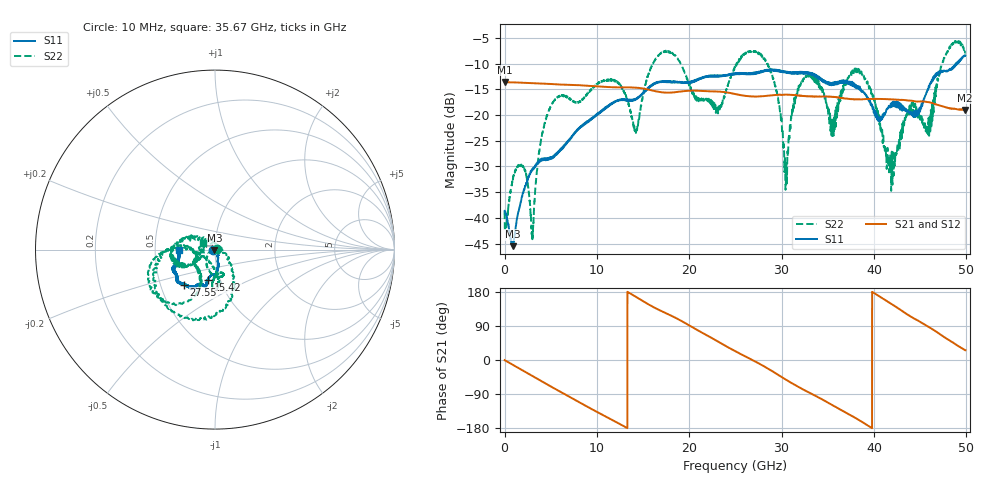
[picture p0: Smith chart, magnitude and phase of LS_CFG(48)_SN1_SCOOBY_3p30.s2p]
!Keysight Technologies,N5245B,MY58422026,A.13.80.08
!Date: Thursday, March 19, 2020 23:41:55
!Correction: S11(Full 2 Port(1,2))
!S21(Full 2 Port(1,2))
!S12(Full 2 Port(1,2))
!S22(Full 2 Port(1,2))
!S2P File: Measurements: S11, S21, S12, S22:
# Hz S DB R 50.0
!freq dBS11 angS11 dBS21 angS21 dBS12 angS12 dBS22 angS22
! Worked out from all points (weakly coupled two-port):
!   4991 points, 10 MHz to 49.91 GHz, reference 50 ohm
!   highest |S21| = -13.58 dB at 10 MHz (marker M1); lowest = -19.0 dB at 49.82 GHz (marker M2)
!   lowest |S11| = -45.5 dB at 870 MHz (marker M3), VSWR 1.01, Z = 49.7 - j0.416 ohm
!   |S11| at or under -10 dB: start of sweep to 48.89 GHz; 48.93533 GHz to 48.99183 GHz (56.5 MHz wide, 0.115 % of centre)
!   |S22| runs from -44.2 to -5.5 dB; largest |S21 - S12| = 0.002
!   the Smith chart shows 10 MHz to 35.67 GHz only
!   S11 on the Smith chart (normalised r, x): 10 MHz: 0.98, -0.01; 15.42 GHz: 0.87, -0.31; 27.55 GHz: 0.66, -0.28; 35.67 GHz: 0.67, -0.00
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1e7  -38.64 -166.1  -13.58 -0.3  -13.57 -0.3  -38.84 3.9
8.7e8  -45.51 -127.8  -13.64 -12.3  -13.64 -12.3  -32.73 -48.1
2.1e9  -34.51 -55.9  -13.71 -29.5  -13.70 -29.5  -30.35 -0.3
3.02e9  -30.75 -55.4  -13.78 -42.2  -13.77 -42.2  -44.15 117.6
4.78e9  -28.34 -64.7  -13.93 -66.6  -13.92 -66.6  -19.24 -112.7
8.33e9  -22.31 -77.5  -14.22 -114.7  -14.21 -114.6  -17.15 -85.4
1.204e10  -17.38 -86.7  -14.60 -163.2  -14.60 -163.2  -13.41 -87.7
1.422e10  -17.02 -97.1  -14.66 166.8  -14.65 166.9  -23.35 -135.1
1.542e10  -15.11 -102.9  -14.98 149.3  -14.98 149.4  -13.04 177.6
1.665e10  -13.64 -104.5  -15.46 133.2  -15.46 133.2  -8.46 -164.4
2.301e10  -12.54 -118.5  -15.42 50.3  -15.42 50.4  -19.47 -163.9
2.496e10  -12.04 -122.9  -15.88 23.5  -15.87 23.7  -10.81 -174.0
2.755e10  -11.62 -131.3  -16.37 -9.2  -16.37 -9.0  -8.09 -102.2
3.048e10  -11.76 -143.9  -16.04 -51.8  -16.05 -51.5  -31.68 43.4
3.149e10  -11.63 -149.9  -16.13 -66.5  -16.14 -66.2  -16.22 148.5
3.328e10  -11.98 -158.0  -16.36 -89.8  -16.36 -89.5  -12.24 -164.9
3.567e10  -13.99 -179.8  -16.47 -121.0  -16.41 -120.6  -22.45 152.8
3.84e10  -14.99 169.3  -16.96 -158.7  -16.91 -159.0  -11.12 -160.4
4.16e10  -18.29 101.1  -16.93 152.5  -16.95 152.4  -28.23 93.7
4.675e10  -11.90 6.2  -17.94 74.9  -17.96 75.1  -14.14 -138.1
4.982e10  -8.48 -17.3  -19.01 26.9  -19.02 27.0  -7.19 -12.8
4.991e10  -8.42 -16.5  -18.99 25.8  -19.01 25.8  -7.80 -13.0
